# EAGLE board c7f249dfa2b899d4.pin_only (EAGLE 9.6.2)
REV: G

Size 50.8 x 22.86 mm. Coordinates in mm from the lower left corner, seen from the top.
Outline: 2.54,0 48.26,0 arc90 50.8,2.54 50.8,20.32 arc90 48.26,22.86 2.54,22.86 arc90 0,20.32 0,13.97 0.51,13.46 0.51,9.53 0,9.02 0,2.54 arc90 2.54,0
Copper layers (1*16): Top 0.035mm / dielectric 1.5mm / Bottom 0.035mm
Design rules "adafruit *": minimum track width 8mil, minimum drill 15.5mil, track to track 8mil, track to pad 8mil, pad to pad 8mil, via to via 8mil, smd to smd 8mil, copper to edge 10mil, drill to drill 8mil, minimum pad ring 10mil, minimum via ring 8mil, stop-mask expansion 2mil, vias tented up to drill 20mil, thermal gap 10mil
Net classes: 1 power: width 0.305 mm; 2 gnd: width 0.254 mm
Holes 2.2 mm at 48.26,1.84 48.26,20.95

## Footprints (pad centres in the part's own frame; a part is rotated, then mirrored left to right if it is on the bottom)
0805_10MGAP = smd 1.2 x 1.5: 1 -1.05,0; 2 1.05,0
0805-NO = smd 1.24 x 1.5: 1 -0.95,0; 2 0.95,0
0603-NO = smd 1.075 x 1: 1 -0.85,0; 2 0.85,0
CHIPLED_0603_NOOUTLINE = smd 0.8 x 0.8: A 0,-0.75; C 0,0.75
SOD-123 = smd 1.4 x 1.4: A 1.85,0; C -1.85,0
QFN24_4MM_SMSC = smd 0.8 x 0.28: 1 -2,1.25; 2 -2,0.75; 3 -2,0.25; 4 -2,-0.25; 5 -2,-0.75; 6 -2,-1.25; 13 2,-1.25; 14 2,-0.75; 15 2,-0.25; 16 2,0.25; 17 2,0.75; 18 2,1.25 | smd 0.28 x 0.8: 7 -1.25,-2; 8 -0.75,-2; 9 -0.25,-2; 10 0.25,-2; 11 0.75,-2; 12 1.25,-2; 19 1.25,2; 20 0.75,2; 21 0.25,2; 22 -0.25,2; 23 -0.75,2; 24 -1.25,2 | smd 2.5 x 2.5: THERM 0,0
1X16_ROUND = drill 1 pad 1.676: 1 -19.05,0; 2 -16.51,0; 3 -13.97,0; 4 -11.43,0; 5 -8.89,0; 6 -6.35,0; 7 -3.81,0; 8 -1.27,0; 9 1.27,0; 10 3.81,0; 11 6.35,0; 12 8.89,0; 13 11.43,0; 14 13.97,0; 15 16.51,0; 16 19.05,0
1X12_ROUND = drill 1 pad 1.676: 1 -13.97,0; 2 -11.43,0; 3 -8.89,0; 4 -6.35,0; 5 -3.81,0; 6 -1.27,0; 7 1.27,0; 8 3.81,0; 9 6.35,0; 10 8.89,0; 11 11.43,0; 12 13.97,0
SOT23-3 = smd 0.8 x 0.9: 1 -0.95,-1; 2 0.95,-1; 3 0,1.1
SOT23-R = smd 0.635 x 1.016: 1 -0.95,-1; 2 0.95,-1; 3 0,1
RESPACK_4X0603_NO = smd 0.45 x 0.9: 1 -1.3,-0.85; 2 -0.4,-0.85; 3 0.4,-0.85; 4 1.3,-0.85; 5 1.3,0.85; 6 0.4,0.85; 7 -0.4,0.85; 8 -1.3,0.85
BTN_KMR2_4.6X2.8 = smd 0.9 x 0.9: A 2.05,0.8; A' -2.05,0.8; B 2.05,-0.8; B' -2.05,-0.8
SOT23-5 = smd 0.55 x 1.2: 1 -0.95,-1.3; 2 0,-1.3; 3 0.95,-1.3; 4 0.95,1.3; 5 -0.95,1.3
MOUNTINGHOLE_2.5_PLATED = drill 2.5 pad 3.2: P$1 0,0
FIDUCIAL_1MM = smd 1 x 1: 1 0,0
JSTPH2_BATT = smd 1 x 4.6: 1 -1,-3.7; 2 1,-3.7 | smd 1.6 x 3.4: NC1 -3.4,1.5; NC2 3.4,1.5
ESP-12F = smd 1.7 x 1.1: 1 -7.65,5.77; 2 -7.65,3.77; 3 -7.65,1.77; 4 -7.65,-0.23; 5 -7.65,-2.23; 6 -7.65,-4.23; 7 -7.65,-6.23; 8 -7.65,-8.23; 9 7.65,-8.23; 10 7.65,-6.23; 11 7.65,-4.23; 12 7.65,-2.23; 13 7.65,-0.23; 14 7.65,1.77; 15 7.65,3.77; 16 7.65,5.77
4UCONN_20329_V2 = smd 1 x 2: BASE@1 -0.75,-2; BASE@2 0.75,-2 | smd 0.4 x 1.35: D+ 0,0.775; D- -0.65,0.775; GND 1.3,0.775; ID 0.65,0.775; VBUS -1.3,0.775 | drill 0.8 pad 1.143 offset: SPRT@1 -3.3,0.9; SPRT@2 3.3,0.9 | drill 0.9 pad 2.413 square: SPRT@3 -3.6,-1.9; SPRT@4 3.6,-1.9 | hole 0.7: -1.95,0; 1.95,0

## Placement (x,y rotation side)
C2  10uF  [0805_10MGAP]  23.88,18.67 180 top
C3  10µF  [0805-NO]  17.59,18.61 0 top
C6  10µF  [0805-NO]  12.36,9.77 270 top
C7  1uF  [0603-NO]  12.78,3.95 180 top
C8  10µF  [0805-NO]  15.67,16.06 90 top
CHG  ORANGE  [CHIPLED_0603_NOOUTLINE]  1.71,5.65 270 top
D3  RED  [CHIPLED_0603_NOOUTLINE]  2.22,17.46 270 top
D4  MBR0540  [SOD-123]  10.41,12.32 180 top
IC1  CP2104  [QFN24_4MM_SMSC]  17.14,6.1 0 top
JP1  [1X16_ROUND]  25.4,1.27 180 top
JP3  [1X12_ROUND]  30.48,21.59 0 top
Q1  mmbt2222  [SOT23-3]  23.94,5.21 180 top
Q2  mmbt2222  [SOT23-3]  24.07,12.32 0 top
Q3  DMG341  [SOT23-R]  9.65,9.91 0 top
R1  10k  [0603-NO]  14.73,9.33 180 top
R2  10K  [RESPACK_4X0603_NO]  24,8.76 90 top
R3  10K  [0603-NO]  9.53,3.94 0 top
R4  100K  [0603-NO]  18.54,12.64 180 top
R7  4.7K  [RESPACK_4X0603_NO]  21.78,16.07 270 top
R11  1K  [0603-NO]  18.29,10.54 0 top
SW2  KMR2  [BTN_KMR2_4.6X2.8]  10.41,6.29 0 top
U2  AP2112-3.3  [SOT23-5]  15.11,12.19 0 top
U3  MCP73831T-2ACI/OT  [SOT23-5]  18.54,15.62 180 top
U$7  [ADAFRUIT_5MM]  45.66,13.91 90 bottom
U$9  [FEATHERLOGO]  30.67,4.89 0 bottom
U$13  [PCBFEAT-REV-040]  4.64,11.24 0 bottom
U$15  [ADAFRUIT_3.5MM]  22.48,7.11 90 top
U$23  [HUZZAHLOGO]  49.91,10.29 0 bottom
U$31  MOUNTINGHOLE2.5  [MOUNTINGHOLE_2.5_PLATED]  2.54,20.32 270 top
U$32  MOUNTINGHOLE2.5  [MOUNTINGHOLE_2.5_PLATED]  2.54,2.54 270 top
U$34  FIDUCIAL_1MM  [FIDUCIAL_1MM]  10.79,20.07 270 top
U$35  FIDUCIAL_1MM  [FIDUCIAL_1MM]  44.88,4.71 270 top
X1  JSTPH  [JSTPH2_BATT]  10.79,19.3 0 top
X3  ESP-12F  [ESP-12F]  36,11.43 270 top
X4  20329  [4UCONN_20329_V2]  4.45,11.43 270 top

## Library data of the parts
C2 C3 C6 C7 CHG D3 D4 IC1 JP1 JP3 Q3 R1-R4 R7 R11 SW2 U2 U3 U$7 U$9 U$13 U$15 U$23 X1 X3 X4 = microbuilder
C8 = microbuilder; COMPANY: ADAFRUIT INDUSTRIES; DRAWN: KTOWN; REV: G
Q1 Q2 = SparkFun
U$31 U$32 U$34 U$35 = microbuilder; BOM: EXCLUDE

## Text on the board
tPlace: 5 | 4 | 14 | 12 | 13 | 15 | 0 | 16 | 2 | BAT | EN | USB | SCL | SDA | #0 | huzzah! | RST | CHG | RST | 3V | NC | GND | ADC | NC | NC | NC | NC | NC | SCK | MO | MI | RX | TX | CHPD
bPlace: 3.7/4.2V / LiPoly Batt / µUSB charge | En | 0 | 2 | BAT | USB | 14 | 12 | 13 | 15 | 16 | SCL/5 | SDA/4 | Feather HUZZAH / ESP8266 WiFi | 4MB Flash / 80MHz & 3.3V | 14/SCK | 13/MOSI | 12/MISO | RST | CHPD | 3V | NC | GND | ADC | NC | NC | NC | NC | NC | RX | TX

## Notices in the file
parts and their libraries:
microbuilder: This work is placed in the public domain, and may be freely used for commercial and non-commercial work with the following conditions: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
SparkFun: Licensing: CC v3.0 Share-Alike You are welcome to use this library for commercial purposes.
